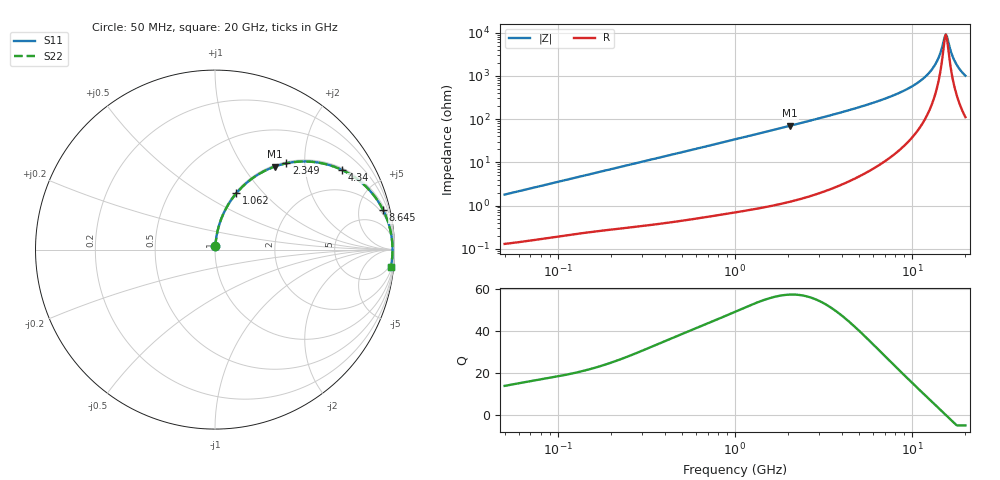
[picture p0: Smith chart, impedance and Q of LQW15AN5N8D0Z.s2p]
!Murata Part Number: LQW15AN5N8D0Z
!These Parameters are Measured in Series Mode Connection
!  o--[Z]--o
!Port1  Port2
!  o-------o
!Freq. Start=50[MHz] Stop=20[GHz], 401[Steps]
# Hz S RI R 50
!Freq.(Hz) S11(Real) S11(Imag) S21(Real) S21(Imag) S12(Real) S12(Imag) S22(Real) S22(Imag)
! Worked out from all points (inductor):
!   401 points, 50 MHz to 20 GHz, reference 50 ohm
!   read as one part in series: L = 5.65 nH near 51.52 MHz
!   highest Q = 57.2 at 2.052 GHz (marker M1), where L = 5.45 nH
!   self-resonance near 15.5 GHz
!   S11 on the Smith chart (normalised r, x): 50 MHz: 1.00, +0.04; 1.062 GHz: 1.01, +0.72; 2.349 GHz: 1.03, +1.62; 4.34 GHz: 1.07, +3.16; 8.645 GHz: 1.41, +8.40; 20 GHz: 3, -20
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5e7  0.00161 0.0178  0.9984 -0.0178  0.9984 -0.0178  0.00161 0.0178
1.364002e8  0.00452 0.0472  0.9955 -0.0472  0.9955 -0.0472  0.00452 0.0472
3.721004e8  0.0195 0.1243  0.9805 -0.1243  0.9805 -0.1243  0.0195 0.1243
1e9  0.1082 0.3006  0.8918 -0.3006  0.8918 -0.3006  0.1082 0.3006
1.061746e9  0.1198 0.3149  0.8802 -0.3149  0.8802 -0.3149  0.1198 0.3149
2.05233e9  0.3333 0.4627  0.6667 -0.4627  0.6667 -0.4627  0.3333 0.4627
2.348516e9  0.3968 0.4805  0.6032 -0.4805  0.6032 -0.4805  0.3968 0.4805
2.728004e9  0.4728 0.4903  0.5272 -0.4903  0.5272 -0.4903  0.4728 0.4903
4.34015e9  0.71 0.4427  0.29 -0.4427  0.29 -0.4427  0.71 0.4427
7.442007e9  0.9044 0.2754  0.0956 -0.2754  0.0956 -0.2754  0.9044 0.2754
8.644534e9  0.9368 0.22  0.0632 -0.22  0.0632 -0.22  0.9368 0.22
1.082228e10  0.9699 0.1355  0.0301 -0.1355  0.0301 -0.1355  0.9699 0.1355
1.257102e10  0.9826 0.0791  0.0174 -0.0791  0.0174 -0.0791  0.9826 0.0791
1.396067e10  0.9875 0.0397  0.0125 -0.0397  0.0125 -0.0397  0.9875 0.0397
1.438523e10  0.9883 0.0284  0.0117 -0.0284  0.0117 -0.0284  0.9883 0.0284
1.504638e10  0.989 0.0115  0.011 -0.0115  0.011 -0.0115  0.989 0.0115
1.550395e10  0.9891 0.00025  0.0109 -0.00025  0.0109 -0.00025  0.9891 0.00025
1.597544e10  0.989 -0.011  0.011 0.011  0.011 0.011  0.989 -0.011
1.696185e10  0.988 -0.0335  0.012 0.0335  0.012 0.0335  0.988 -0.0335
1.774144e10  0.9866 -0.0504  0.0134 0.0504  0.0134 0.0504  0.9866 -0.0504
1.88369e10  0.9838 -0.073  0.0162 0.073  0.0162 0.073  0.9838 -0.073
2e10  0.9799 -0.0956  0.0201 0.0956  0.0201 0.0956  0.9799 -0.0956
